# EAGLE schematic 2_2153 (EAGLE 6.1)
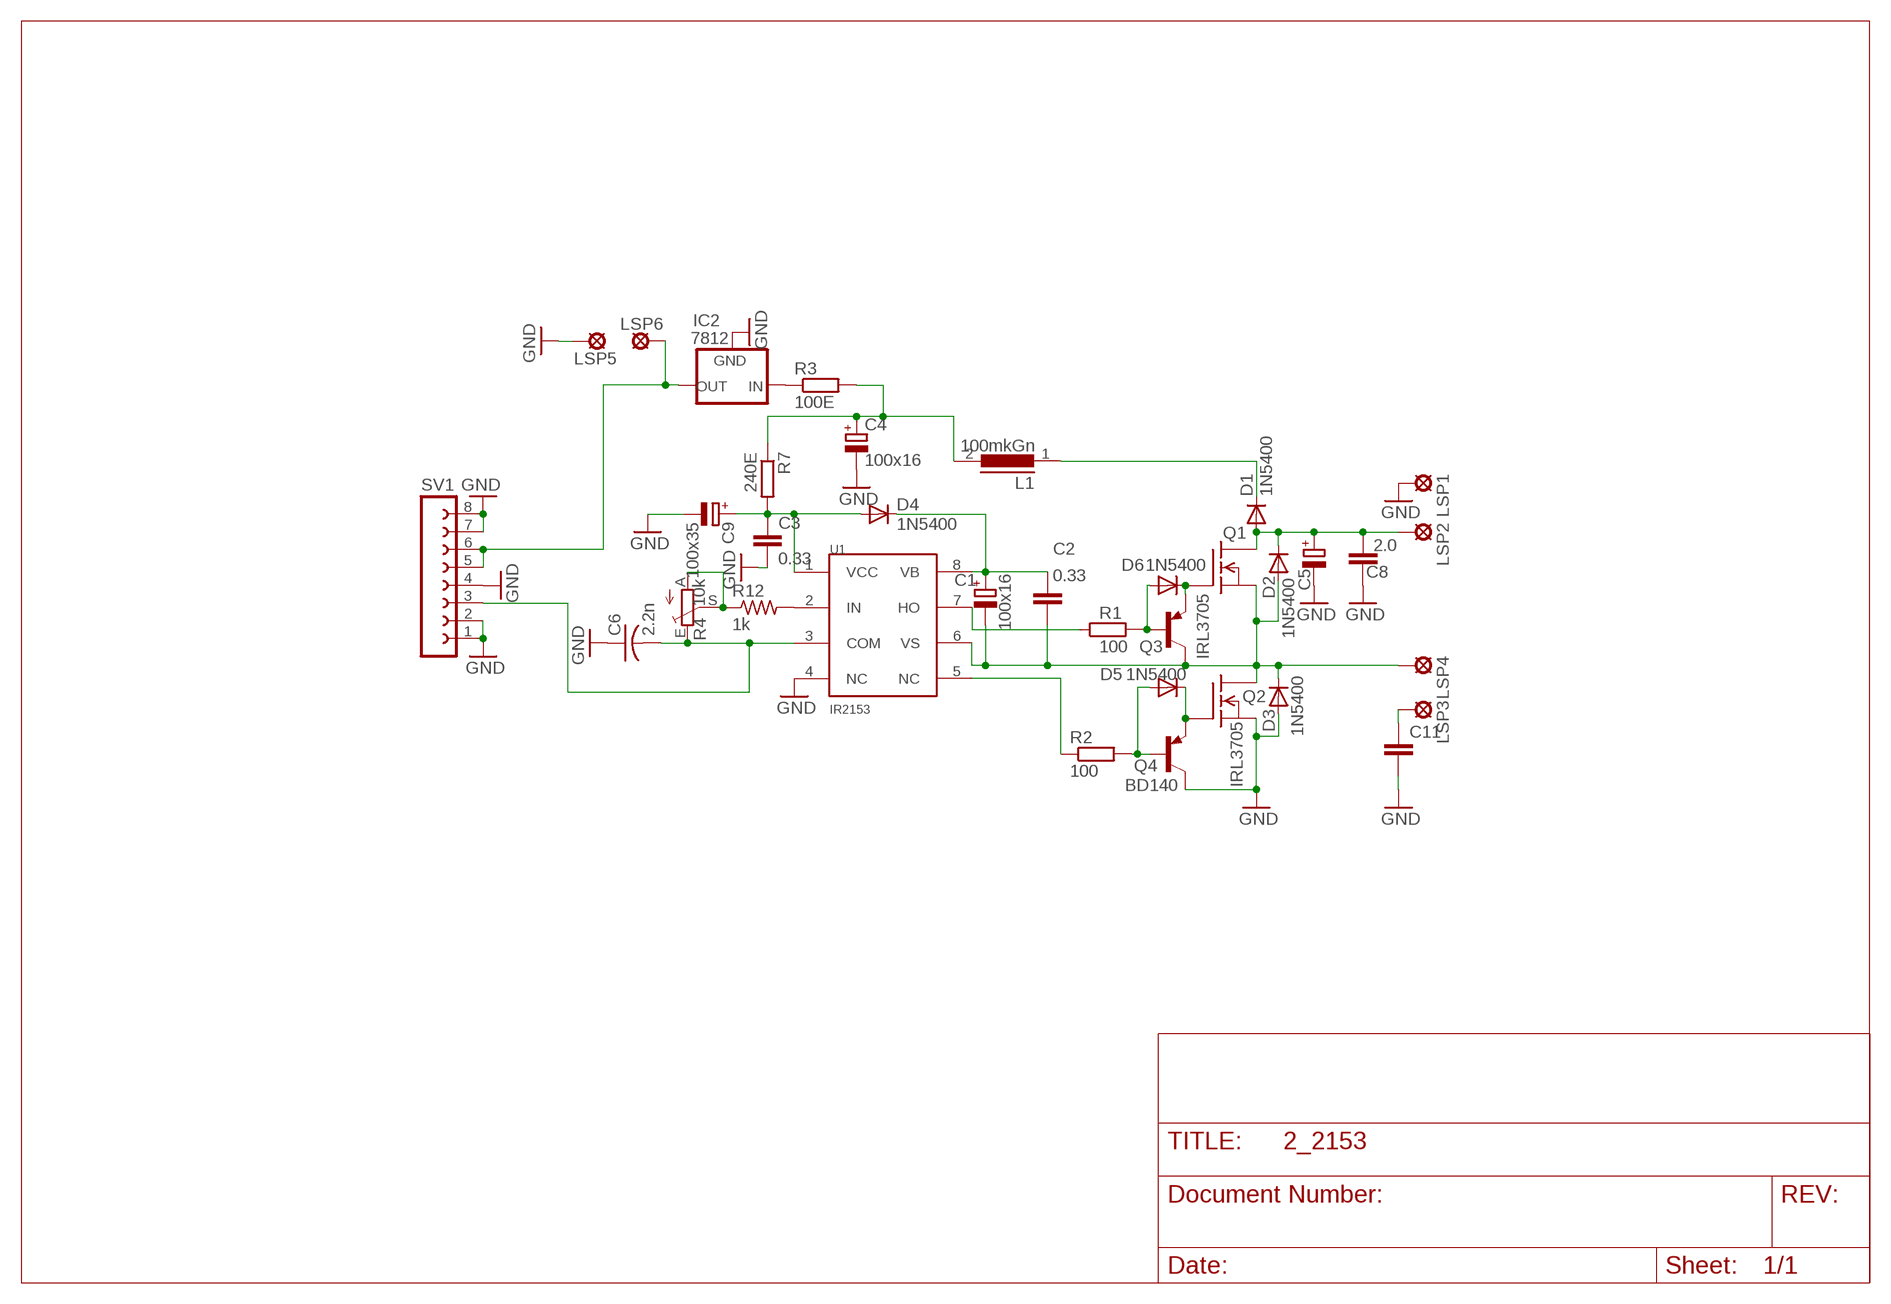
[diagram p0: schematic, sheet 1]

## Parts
C1  100x16  CPOL-EUE3.5-8  [E3,5-8]
C2  0.33  C-EU050-050X075  [C050-050X075]
C3  0.33  C-EU050-050X075  [C050-050X075]
C4  100x16  CPOL-EUE3.5-8  [E3,5-8]
C5  CPOL-EUE10-25  [EB25D]
C6  2.2n  C-US050-035X075  [C050-035X075]
C8  2.0  C-EU150-091X182  [C150-091X182]
C9  100x35  CPOL-EUE3.5-8  [E3,5-8]
C11  C-EU375-203X418  [C375-203X418]
D1  1N5400  [DO201-15]
D2  1N5400  [DO201-15]
D3  1N5400  [DO201-15]
D4  1N5400  [DO201-15]
D5  1N5400  [DO201-15]
D6  1N5400  [DO201-15]
IC2  7812  LP2950CDT-3.3  [DPACK]
L1  100mkGn  82114R  [82114R]
LSP1  MCS10B  [MCS10B]
LSP2  MCS10B  [MCS10B]
LSP3  MCS10B  [MCS10B]
LSP4  MCS10B  [MCS10B]
LSP5  MCS10B  [MCS10B]
LSP6  MCS10B  [MCS10B]
Q1  IRL3705  IRF840  [TO220]
Q2  IRL3705  IRF840  [TO220]
Q3  BD140  [TO126]
Q4  BD140  [TO126]
R1  100  R-EU_0613/15  [P0613/15]
R2  100  R-EU_0613/15  [P0613/15]
R3  100E  R-EU_0613/15  [P0613/15]
R4  10k  TRIM_EU-CA6V  [CA6V]
R7  240E  R-EU_0613/15  [P0613/15]
R12  1k  R-US_0207/12  [0207/12]
SV1  FE08-1  [FE08]
U1  IR2153  IR2117  [DIL08]

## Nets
COM: C6.2 R4.E SV1.3 U1.3(COM)
GND: C3.2 C4.- C5.- C6.1 C8.1 C9.- C11.2 D3.A IC2.4(GND) LSP1.MP LSP5.MP Q2.3(S) Q4.2(C) SV1.1 SV1.2 SV1.4 SV1.7 SV1.8 U1.4(NC)
N$1: D6.A Q3.3(B) R1.2
N$2: R12.2 U1.2(IN)
N$3: D5.A Q4.3(B) R2.2
N$4: C4.+ L1.2 R3.2 R7.1
N$5: R1.1 U1.7(HO)
N$6: R4.A R4.S R12.1
N$7: IC2.3(OUT) LSP6.MP SV1.5 SV1.6
N$8: R2.1 U1.5(NC)
N$9: IC2.1(IN) R3.1
N$10: D5.C Q2.1(G) Q4.1(E)
N$11: D6.C Q1.1(G) Q3.1(E)
N$13: D1.C L1.1
N$19: C11.1 LSP3.MP
N$22: C5.+ C8.2 D1.A D2.C LSP2.MP Q1.2(D)
VB: C1.+ C2.1 D4.C U1.8(VB)
VCC: C3.1 C9.+ D4.A R7.2 U1.1(VCC)
VS: C1.- C2.2 D2.A D3.C LSP4.MP Q1.3(S) Q2.2(D) Q3.2(C) U1.6(VS)

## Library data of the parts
C1 C4 C5 C9 = rcl:CPOL-EU: POLARIZED CAPACITOR, European symbol
C2 C3 C8 C11 = rcl:C-EU: CAPACITOR, European symbol
C6 = rcl:C-US: CAPACITOR, American symbol
D1-D6 = diode:1N5400: DIODE
IC2 = v-reg:LP2950?*: Source: http://cache.national.com/ds/LP/LP2950.pdf
L1 = inductors:82114R: INDUCTOR
LSP1-LSP6 = solpad:MCS10B: SOLDER PAD
Q1 Q2 = transistor-fet:IRF840: N-Channel Enhancement MOSFET (HEXFET); 500V; 8A; 0,85Ohm
Q3 Q4 = transistor-pnp:BD140: PNP Transistor
R1-R3 R7 = rcl:R-EU_: RESISTOR, European symbol
R4 = pot:TRIM_EU-: POTENTIOMETER
R12 = rcl:R-US_: RESISTOR, American symbol
SV1 = con-lsta:FE08-1: FEMALE HEADER
U1 = irf:IR2117: High side driver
